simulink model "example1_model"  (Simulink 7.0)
settings: Solver=ode45  StartTime=0.0  StopTime=10.0  RelTol=1e-3
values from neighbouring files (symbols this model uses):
  Ccit_Z = pol2mat(Ccit_Zp)    [example_3_6_1_podklad.m]    (also in example_3_6_3_podklad.m)
  Cjmn_Z = pol2mat(Cjmn_Zp)    [example_3_6_1_podklad.m]    (also in example_3_6_2_podklad.m; example_3_6_3_podklad.m)

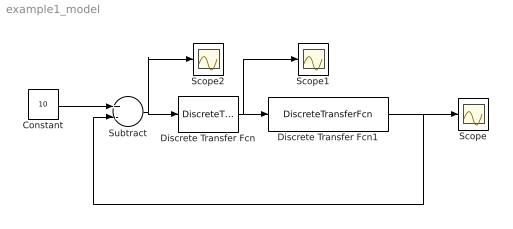
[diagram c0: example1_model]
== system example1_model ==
  Constant : Constant  Value=10  OutDataType=sfix(16)  OutScaling=2^0
  Discrete Transfer Fcn : DiscreteTransferFcn  Numerator=Ccit_Z  Denominator=Cjmn_Z
  Discrete Transfer Fcn1 : DiscreteTransferFcn  Numerator=[1 -3.5 -2]  Denominator=[1 -3.5 3.5 -1]
  Scope : Scope
  Scope1 : Scope
  Scope2 : Scope
  Subtract : Sum  Inputs=+-  OutDataType=sfix(16)  OutScaling=2^-10
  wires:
  Constant/1 -> Subtract/1
  Subtract/1 -> Discrete Transfer Fcn/1, Scope2/1
  Discrete Transfer Fcn/1 -> Discrete Transfer Fcn1/1, Scope1/1
  Discrete Transfer Fcn1/1 -> Subtract/2, Scope/1
